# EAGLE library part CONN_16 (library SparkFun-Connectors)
Multi connection point. Often used as Generic Header-pin footprint for 0.1 inch spaced/style header connections On any of the 0.1 inch spaced packages, you can populate with these: Break Away Headers - Straight (PRT-00116) Break Away Male Headers - Right Angle (PRT-00553) Female Headers (PRT-00115) Break Away Headers - Machine Pin (PRT-00117) Break Away Female Headers - Swiss Machine Pin (PRT-00743) For SCREWTERMINALS and SPRING TERMINALS visit here: Screw Terimnals on SparkFun.com (5mm/3.5mm/2.54mm spacing) This device is also useful as a general connection point to wire up your design to another part of your project. Our various solder wires solder well into these plated through hole pads. Hook-Up Wire - Assortment (Stranded, 22 AWG) (PRT-11375) Hook-Up Wire - Assortment (Solid Core, 22 AWG) (PRT-11367) View the entire wire category on our website here Special notes: Molex polarized connector foot print use with SKU : PRT-08231 with associated crimp pins and housings. 1MM SMD Version SKU: PRT-10208 NOTES ON THE VARIANTS LOCK and LOCK_LONGPADS... This footprint was designed to help hold the alignment of a through-hole component (i.e. 6-pin header) while soldering it into place. You may notice that each hole has been shifted either up or down by 0.005 of an inch from it's more standard position (which is a perfectly straight line). This slight alteration caused the pins (the squares in the middle) to touch the edges of the holes. Because they are alternating, it causes a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
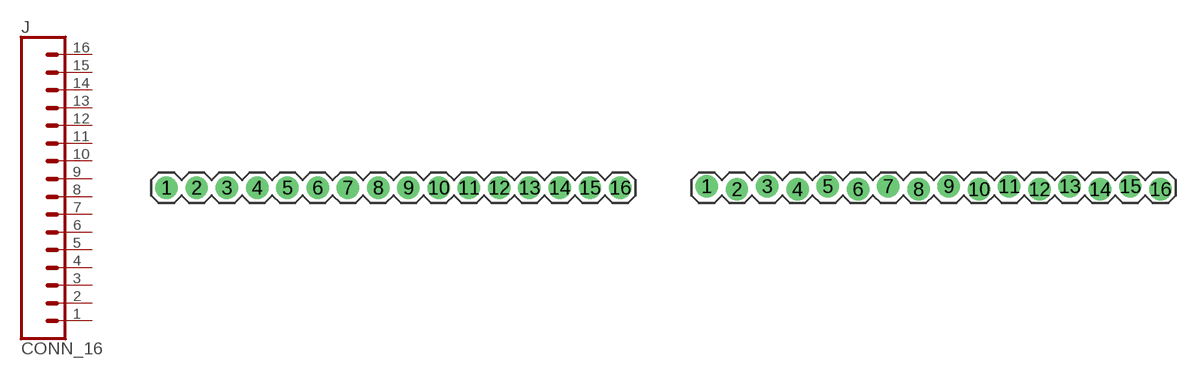
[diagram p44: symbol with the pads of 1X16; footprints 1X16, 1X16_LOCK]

Designator prefix J

## CONN_16  [1X16]
1  1  pas
2  2  pas
3  3  pas
4  4  pas
5  5  pas
6  6  pas
7  7  pas
8  8  pas
9  9  pas
10  10  pas
11  11  pas
12  12  pas
13  13  pas
14  14  pas
15  15  pas
16  16  pas

## CONN_16LOCK  [1X16_LOCK]
Pads as for 1X16

## CONN_16LOCK_LONGPADS  [1X16_LOCK_LONGPADS]
Pads as for 1X16

## CONN_16MACHIINE-PIN_LOCK  [1X16_MACHINE-PIN-HEADER_LOCK.004]
Pads as for 1X16

## CONN_16LONGPADS  [1X16_LONGPADS]
Pads as for 1X16

## CONN_161X16_NO_SILK  [1X16_NO_SILK]
Pads as for 1X16

## CONN_161X16_SM_SQ_NOSILK  [1X16_SM_SQ_NOSILK]
Pads as for 1X16

## Footprint 1X16 (pad centres in mm)
Plated Through Hole -16 Pin Specifications: Pin count:16 Pin pitch:0.1" Example device(s): CONN_16
drill 1.016 pad 1.88: 1 0,0; 2 2.54,0; 3 5.08,0; 4 7.62,0; 5 10.16,0; 6 12.7,0; 7 15.24,0; 8 17.78,0; 9 20.32,0; 10 22.86,0; 11 25.4,0; 12 27.94,0; 13 30.48,0; 14 33.02,0; 15 35.56,0; 16 38.1,0

## Footprint 1X16_LOCK (pad centres in mm)
Plated Through Hole -16 Pin Locking Footprint Holes are offset 0.005" to hold pins in place while soldering. Specifications: Pin count:16 Pin pitch:0.1" Example device(s): CONN_16
drill 1.016 pad 1.88: 1 0,0.127; 2 2.54,-0.127; 3 5.08,0.127; 4 7.62,-0.127; 5 10.16,0.127; 6 12.7,-0.127; 7 15.24,0.127; 8 17.78,-0.127; 9 20.32,0.127; 10 22.86,-0.127; 11 25.4,0.127; 12 27.94,-0.127; 13 30.48,0.127; 14 33.02,-0.127; 15 35.56,0.127; 16 38.1,-0.127

## Footprint 1X16_LOCK_LONGPADS (pad centres in mm)
Plated Through Hole -16 Pin Locking Footprint w/ Long Pads Holes are offset 0.005" to hold pins in place while soldering. Specifications: Pin count:16 Pin pitch:0.1" Example device(s): CONN_16
drill 1.016 long: 1 0,0.127; 2 2.54,-0.127; 3 5.08,0.127; 4 7.62,-0.127; 5 10.16,0.127; 6 12.7,-0.127; 7 15.24,0.127; 8 17.78,-0.127; 9 20.32,0.127; 10 22.86,-0.127; 11 25.4,0.127; 12 27.94,-0.127; 13 30.48,0.127; 14 33.02,-0.127; 15 35.56,0.127; 16 38.1,-0.127

## Footprint 1X16_MACHINE-PIN-HEADER_LOCK.004 (pad centres in mm)
Plated Through Hole -16 Pin Machine Pin Header Locking Footprint Holes are offset 0.005" to hold pins in place while soldering. Specifications: Pin count:16 Pin pitch:0.1" Example device(s): CONN_16
drill 0.889: 1 0,0.102; 2 2.54,-0.102; 3 5.08,0.102; 4 7.62,-0.102; 5 10.16,0.102; 6 12.7,-0.102; 7 15.24,0.102; 8 17.78,-0.102; 9 20.32,0.102; 10 22.86,-0.102; 11 25.4,0.102; 12 27.94,-0.102; 13 30.48,0.102; 14 33.02,-0.102; 15 35.56,0.102; 16 38.1,-0.102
